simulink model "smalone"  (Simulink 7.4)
settings: Solver=ode23t  StartTime=0.0  StopTime=10  MaxStep=0.001  RelTol=1e-5  AbsTol=1e-4
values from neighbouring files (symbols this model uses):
  Ef = parEf(m)    [Ccurverun.m]
  Ra = .95    (= 0.95)    [altwdgs.m]    (also in Ccurverun.m = 0.018)
  wo = 2*pi*freq0    [calc0.m]    (also in IMabc2.m = 376.991118431; imabcparam.m = 376.991118431; IMabcrun0.m = 376.991118431; IMabcrun1.m = 376.991118431)
undefined symbols (not defined in the file or in its folder): fa0, fk0, Lal, Lfl, Lkdl, Lkql, Lload, Lmd, Lmq, phif0, Rf, Rkd, Rkq, Rload, vf0

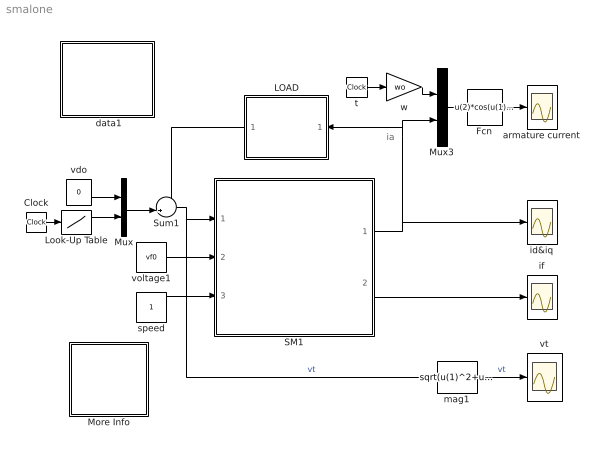
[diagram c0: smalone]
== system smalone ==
  note: ia
  " data1" : Subsystem
  Clock : Clock
  Fcn : Fcn  Expr=u(2)*cos(u(1))-u(3)*sin(u(1))
  LOAD : Subsystem
  Look-Up Table : Lookup  InputValues=[0 0.5 0.51 20]  Table=[Ef Ef 0 0]  OutDataType=sfix(16)  OutScaling=2^0
  More Info : Subsystem
  Mux : Mux  Inputs=2
  Mux3 : Mux  Inputs=2
  SM1 : Subsystem
  Sum1 : Sum  Inputs=-+|  OutDataType=sfix(16)  OutScaling=2^0
  armature current : Scope
  id&iq : Scope
  if : Scope
  mag1 : Fcn  Expr=sqrt(u(1)^2+u(2)^2)
  speed : Constant  OutDataType=sfix(16)  OutScaling=2^0
  t : Clock
  vdo : Constant  Value=0  OutDataType=sfix(16)  OutScaling=2^0
  voltage1 : Constant  Value=vf0  OutDataType=sfix(16)  OutScaling=2^0
  vt : Scope
  w : Gain  Gain=wo  ParameterDataType=sfix(16)  ParameterScaling=2^0  OutDataType=sfix(16)  OutScaling=2^0
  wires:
  voltage1/1 -> SM1/2(vf)
  SM1/2(if) -> if/1
  speed/1 -> SM1/3(wm)
  Look-Up Table/1 -> Mux/2
  Mux/1 -> Sum1/2
  Sum1/1 -> SM1/1(vs), mag1/1  "vt"
  SM1/1(ia) -> id&iq/1, LOAD/1("i_in "), Mux3/2
  mag1/1 -> vt/1  "vt"
  vdo/1 -> Mux/1
  Clock/1 -> Look-Up Table/1
  LOAD/1(v_out) -> Sum1/1
  Mux3/1 -> Fcn/1
  Fcn/1 -> armature current/1
  t/1 -> w/1
  w/1 -> Mux3/1

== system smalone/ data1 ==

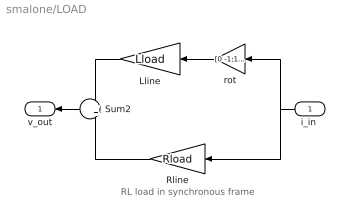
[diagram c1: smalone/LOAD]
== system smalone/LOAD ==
  note: RL load in synchronous frame
  "i_in " : Inport  OutDataType=sfix(16)  OutScaling=2^0
  Lline : Gain  Gain=Lload  ParameterDataType=sfix(16)  ParameterScaling=2^0  OutDataType=sfix(16)  OutScaling=2^0
  Rline : Gain  Gain=Rload  ParameterDataType=sfix(16)  ParameterScaling=2^0  OutDataType=sfix(16)  OutScaling=2^0
  Sum2 : Sum  OutDataType=sfix(16)  OutScaling=2^0
  rot : Gain  Gain=[0 -1;1 0]  Multiplication=Matrix(K*u)  ParameterDataType=sfix(16)  ParameterScaling=2^0  OutDataType=sfix(16)  OutScaling=2^0
  v_out : Outport
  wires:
  "i_in "/1 -> rot/1, Rline/1
  rot/1 -> Lline/1
  Lline/1 -> Sum2/1
  Rline/1 -> Sum2/2
  Sum2/1 -> v_out/1

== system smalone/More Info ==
  note: The generator runs under open-cicuit conditions when an inductive-resistive load is suddenly applied. The model is simplified by assuming constant synchronous speed operation.
  note: Synchronous generator voltage dip
  note: y

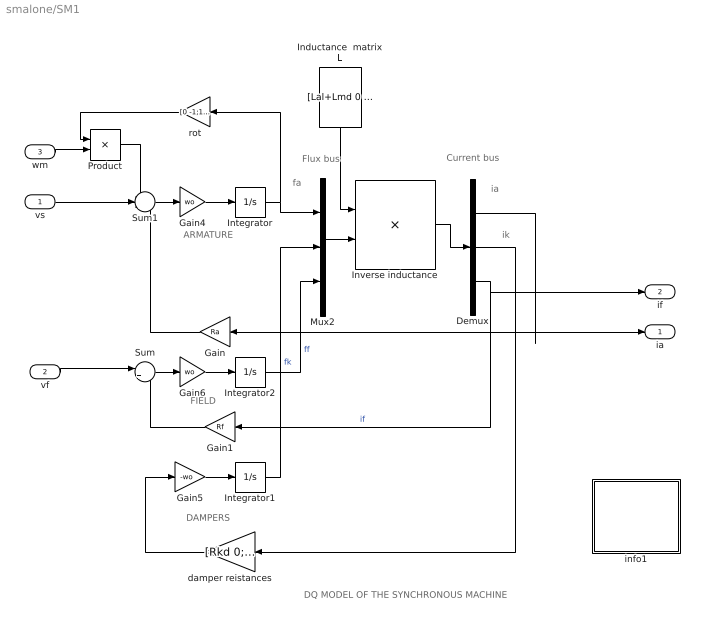
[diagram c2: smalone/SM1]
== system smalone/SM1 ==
  note: DAMPERS
  note: ARMATURE
  note: fa
  note: ia
  note: FIELD
  note: DQ MODEL OF THE SYNCHRONOUS MACHINE
  note: Flux bus
  note: Current bus
  note: ik
  vs : Inport  OutDataType=sfix(16)  OutScaling=2^0
  vf : Inport  Port=2  OutDataType=sfix(16)  OutScaling=2^0
  wm : Inport  Port=3  OutDataType=sfix(16)  OutScaling=2^0
  Demux : Demux  Outputs=3
  Gain : Gain  Gain=Ra  ParameterDataType=sfix(16)  ParameterScaling=2^0  OutDataType=sfix(16)  OutScaling=2^0
  Gain1 : Gain  Gain=Rf  ParameterDataType=sfix(16)  ParameterScaling=2^0  OutDataType=sfix(16)  OutScaling=2^0
  Gain4 : Gain  Gain=wo  ParameterDataType=sfix(16)  ParameterScaling=2^0  OutDataType=sfix(16)  OutScaling=2^0
  Gain5 : Gain  Gain=-wo  ParameterDataType=sfix(16)  ParameterScaling=2^0  OutDataType=sfix(16)  OutScaling=2^0
  Gain6 : Gain  Gain=wo  ParameterDataType=sfix(16)  ParameterScaling=2^0  OutDataType=sfix(16)  OutScaling=2^0
  Inductance  matrix L : Constant  Value=[Lal+Lmd 0 Lmd 0 Lmd;0 Lal+Lmq 0 Lmq 0;Lmd 0 Lmd+Lkdl 0 Lmd;0 Lmq 0 Lmq+Lkql 0;Lmd 0 Lmd 0 Lmd+Lfl]  VectorParams1D=off  OutDataType=fixdt(1, 16)  OutScaling=2^0
  Integrator : Integrator  InitialCondition=fa0
  Integrator1 : Integrator  InitialCondition=fk0
  Integrator2 : Integrator  InitialCondition=phif0
  Inverse inductance : Product  Inputs=/*  Multiplication=Matrix(*)  OutDataType=sfix(16)  OutScaling=2^0
  Mux2 : Mux  Inputs=3
  Product : Product  OutDataType=sfix(16)  OutScaling=2^0
  Sum : Sum  Inputs=|+-  OutDataType=sfix(16)  OutScaling=2^0
  Sum1 : Sum  Inputs=-+-  OutDataType=sfix(16)  OutScaling=2^0
  damper reistances : Gain  Gain=[Rkd 0;0 Rkq]  Multiplication=Matrix(K*u)  ParameterDataType=sfix(16)  ParameterScaling=2^0  OutDataType=sfix(16)  OutScaling=2^0
  info1 : Subsystem
  rot : Gain  Gain=[0 -1;1 0]  Multiplication=Matrix(K*u)  ParameterDataType=sfix(16)  ParameterScaling=2^0  OutDataType=sfix(16)  OutScaling=2^0
  ia : Outport
  if : Outport  Port=2
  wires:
  Product/1 -> Sum1/1
  rot/1 -> Product/1
  wm/1 -> Product/2
  Gain5/1 -> Integrator1/1
  damper reistances/1 -> Gain5/1
  Integrator/1 -> Mux2/1, rot/1
  Sum1/1 -> Gain4/1
  Gain4/1 -> Integrator/1
  vs/1 -> Sum1/2
  Gain/1 -> Sum1/3
  Gain6/1 -> Integrator2/1
  Sum/1 -> Gain6/1
  vf/1 -> Sum/1
  Gain1/1 -> Sum/2
  Demux/1 -> Gain/1, ia/1
  Integrator1/1 -> Mux2/2  "fk"
  Integrator2/1 -> Mux2/3  "ff"
  Demux/2 -> damper reistances/1
  Demux/3 -> if/1, Gain1/1  "if"
  Mux2/1 -> Inverse inductance/2
  Inverse inductance/1 -> Demux/1
  Inductance  matrix L/1 -> Inverse inductance/1

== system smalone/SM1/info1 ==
  note: Synchronous machine transients under shortcircuit
  note: This demonstration illustrates the dynamics of a synchronous generator, initially at no load, following a three-phase short circuit at the terminals.
